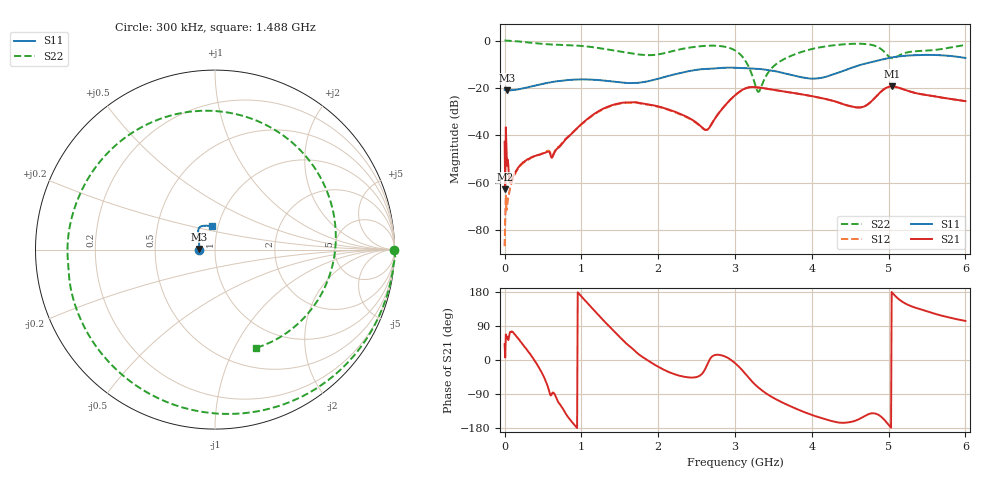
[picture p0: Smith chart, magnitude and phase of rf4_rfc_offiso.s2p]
!Agilent Technologies,M9375A,MY55441453,A.02.50.04
!Agilent M9375A: A.02.50.04
!Date: Monday, December 12, 2016 11:29:29
!Correction: S11(Full 2 Port(1,2))
!S21(Full 2 Port(1,2))
!S12(Full 2 Port(1,2))
!S22(Full 2 Port(1,2))
!S2P File: Measurements: S11, S21, S12, S22:
# Hz S  dB  R 50
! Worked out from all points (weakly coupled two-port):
!   751 points, 300 kHz to 6 GHz, reference 50 ohm
!   highest |S21| = -19.34 dB at 5.04 GHz (marker M1); lowest = -62.8 dB at 8.3 MHz (marker M2)
!   lowest |S11| = -21.1 dB at 32.3 MHz (marker M3), VSWR 1.19, Z = 41.9 + j0.304 ohm
!   |S11| at or under -10 dB: start of sweep to 4.664 GHz
!   |S22| runs from -21.7 to 0.0 dB; largest |S21 - S12| = 0.014
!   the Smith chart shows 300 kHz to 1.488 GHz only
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300000  -20.81 -177.2  -42.73 41.8  -86.82 69.1  -0.03 -0.2
8299600  -20.89 179.7  -62.84 6.4  -75.45 97.8  0.05 -2.4
3.22984e7  -21.08 177.7  -52.82 62.1  -70.00 85.4  -0.04 -9.7
8.82956e7  -20.98 170.7  -59.08 75.3  -60.46 81.1  -0.15 -26.0
2.80286e8  -19.90 152.2  -50.60 30.0  -50.76 27.7  -0.70 -82.6
5.60272e8  -17.86 136.6  -46.92 -68.4  -46.61 -72.1  -1.57 -162.6
7.522624e8  -16.89 130.5  -43.40 -126.4  -43.15 -127.5  -1.83 149.1
1.00025e9  -16.40 123.5  -35.27 167.7  -35.40 168.1  -2.27 87.5
1.264237e9  -16.80 113.1  -29.08 109.5  -29.32 110.9  -3.35 8.6
1.520224e9  -17.71 94.7  -26.32 56.4  -26.48 57.8  -4.71 -78.3
1.768212e9  -17.72 70.3  -26.42 11.8  -26.55 13.0  -5.95 -159.7
2.0002e9  -16.11 48.2  -27.80 -17.7  -27.95 -16.9  -5.83 123.1
2.560172e9  -12.12 26.5  -36.37 -38.5  -36.53 -36.2  -2.36 8.2
3.00015e9  -11.49 28.1  -23.10 -8.1  -23.16 -7.7  -4.16 -70.0
3.304135e9  -11.94 30.3  -19.79 -72.6  -19.82 -72.0  -21.68 121.7
3.60012e9  -13.48 25.2  -21.34 -110.6  -21.34 -110.0  -8.54 -32.1
4.0001e9  -16.09 -7.1  -23.46 -144.9  -23.48 -144.6  -3.58 -103.2
4.688066e9  -9.80 -57.2  -27.73 -147.8  -27.73 -147.5  -1.43 -153.5
5.00005e9  -7.38 -55.0  -19.55 -170.8  -19.57 -170.6  -6.66 -173.3
5.040048e9  -7.11 -54.8  -19.34 179.4  -19.36 179.7  -7.45 -165.7
5.464027e9  -6.03 -49.0  -22.85 130.8  -22.86 131.0  -4.29 166.1
6e9  -7.34 -41.5  -25.56 103.1  -25.58 103.2  -1.87 98.8
